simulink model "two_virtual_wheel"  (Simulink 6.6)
settings: Solver=ode45  StartTime=0.0  StopTime=tfinal  FixedStep=Deltat  RelTol=1e-3
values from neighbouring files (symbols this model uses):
  Jw1 = .5*1.5/4    (= 0.1875)    [two_virtual_wheel_params.m]    (also in two_virtual_wheels.m)
  Jw2 = .5*.015/4    (= 0.001875)    [two_virtual_wheel_params.m]    (also in two_virtual_wheels.m)
  k1 = .5*15    (= 7.5)    [two_virtual_wheel_params.m]    (also in two_virtual_wheels.m)
  k2 = .5*15    (= 7.5)    [two_virtual_wheel_params.m]    (also in two_virtual_wheels.m)
  step_time = 1    [two_virtual_wheel_params.m]    (also in two_virtual_wheels.m)
  Theta_z_0 = 45    [two_virtual_wheel_params.m]    (also in two_virtual_wheels.m)

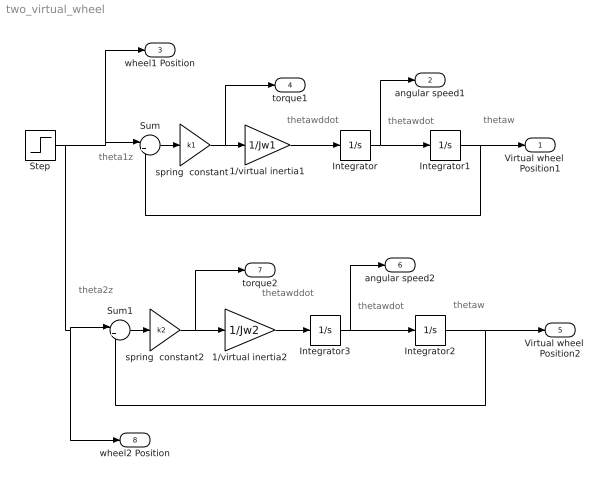
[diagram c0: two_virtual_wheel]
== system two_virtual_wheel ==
  note: thetaw
  note: thetawdot
  note: thetawddot
  note: theta1z
  note: thetaw
  note: thetawdot
  note: thetawddot
  note: theta2z
  1/virtual inertia1 : Gain  Gain=1/Jw1
  1/virtual inertia2 : Gain  Gain=1/Jw2
  Integrator{,1..3} (4 alike) : Integrator
  Step : Step  Time=step_time  After=Theta_z_0  SampleTime=0
  Sum : Sum  Inputs=|+-
  Sum1 : Sum  Inputs=|+-
  spring  constant1 : Gain  Gain=k1
  spring  constant2 : Gain  Gain=k2
  Virtual wheel     Position1 : Outport
  angular speed1 : Outport  Port=2
  wheel1 Position : Outport  Port=3
  torque1 : Outport  Port=4
  Virtual wheel     Position2 : Outport  Port=5
  angular speed2 : Outport  Port=6
  torque2 : Outport  Port=7
  wheel2 Position : Outport  Port=8
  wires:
  Integrator1/1 -> Virtual wheel     Position1/1, Sum/2
  Sum/1 -> spring  constant1/1
  Step/1 -> wheel1 Position/1, Sum/1, Sum1/1, wheel2 Position/1
  spring  constant1/1 -> 1/virtual inertia1/1, torque1/1
  1/virtual inertia1/1 -> Integrator/1
  Integrator/1 -> angular speed1/1, Integrator1/1
  Integrator2/1 -> Sum1/2, Virtual wheel     Position2/1
  Sum1/1 -> spring  constant2/1
  spring  constant2/1 -> 1/virtual inertia2/1, torque2/1
  1/virtual inertia2/1 -> Integrator3/1
  Integrator3/1 -> angular speed2/1, Integrator2/1
